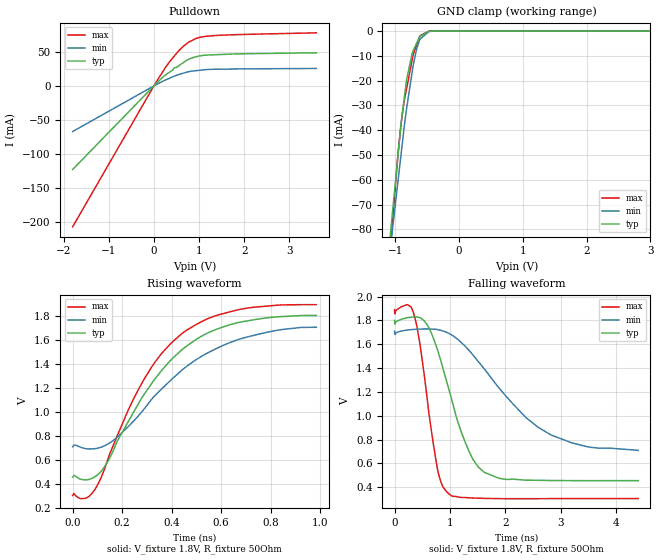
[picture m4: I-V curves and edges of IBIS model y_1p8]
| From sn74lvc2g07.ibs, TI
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|   y_1p8 Model
[Model]   y_1p8
Model_type   Open_drain
Polarity   Non-Inverting
Vmeas = 0.9
Vref = 1.8
Cref = 2pF
Rref = 1200
|   typ   min   max
|   (nom PVT)   (fast PVT)   (slow PVT)
|C_comp from frequency sweep method (F=5MHz)
C_comp   3.504e-12   3.501e-12   3.508e-12
|ON state : BUFFER OUTPUT TURNED LOW
|C_comp   7.638e-12   7.615e-12   7.652e-12
|OFF state: BUFFER IN HIGH IMPEDANCE
|C_comp   3.504e-12   3.501e-12   3.508e-12
|C_comp from LC tank measurement(L=1nH)
|Resonant Frequency(Hz)   2.600e+09   2.640e+09   2.500e+09
|C_comp   3.751e-12   3.638e-12   4.057e-12
|ON state : BUFFER OUTPUT TURNED LOW
|Resonant Frequency(Hz)   2.600e+09   2.640e+09   2.500e+09
|C_comp   3.751e-12   3.638e-12   4.057e-12
|OFF state: BUFFER IN HIGH IMPEDANCE
|Resonant Frequency(Hz)   2.720e+09   2.730e+09   2.710e+09
|C_comp   3.427e-12   3.402e-12   3.452e-12
| Where nom  PVT is Nominal Process, 1.8V, 27C
|   Fast PVT is Strong Process,  1.89V, -40C
|   Slow PVT is Weak Process,   1.71V, 125C
[Voltage Range]   1.8   1.71   1.89
|Ambient Temperature   25   85   -40
|Junction Temperature
[Temperature Range]   27   125   -40
[Pullup Reference]   1.8   1.71   1.89
[Pulldown Reference]   0   0   0
[Power Clamp Reference]   1.8   1.71   1.89
[GND Clamp Reference]   0   0   0
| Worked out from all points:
|   slope of the pulldown table from 0 to 0.27 V, typ, clamps not added: 16.1 ohm
|   GND clamp passes 1 mA (typ) near -0.53 V on its own axis
|   falling waveform, V_fixture 1.8V, R_fixture 50Ohm: 20-80 % time 533ps typ, 1.16ns min, 282ps max; typ from 1.8 V to 0.456 V
|   rising waveform, V_fixture 1.8V, R_fixture 50Ohm: 20-80 % time 278ps typ, 320ps min, 255ps max; typ from 0.457 V to 1.8 V
[Pulldown]
|   Voltage   I(typ)   I(min)   I(max)
-1.8V     -123mA     -67.12mA   -207.3mA
39.69mV   2.626mA    1.43mA     4.492mA
252mV     15.91mA    8.562mA    26.61mA
332.6mV   19.61mA    10.94mA    34.17mA
413.8mV   23.33mA    13.33mA    40.81mA
457.3mV   26.85mA    14.45mA    44.37mA
494.2mV   27.02mA    15.4mA     47.39mA
655.8mV   34.44mA    18.86mA    58.44mA
736.2mV   38.12mA    20.41mA    62.66mA
937.4mV   42.99mA    22.45mA    69.99mA
1.157V    45.34mA    24mA       73.05mA
3.6V      48.76mA    25.7mA     78.1mA
[GND Clamp]
|   Voltage   I(typ)   I(min)   I(max)
-1.8V     -317.6mA   -268.9mA   -375.6mA
-1.067V   -80.12mA   -85.85mA   -86.06mA
-958.2mV  -50.93mA   -61.3mA    -50.42mA
-907.2mV  -37.39mA   -49.82mA   -37.49mA
-863.7mV  -28.48mA   -40.04mA   -29.09mA
-820.8mV  -19.67mA   -31.39mA   -23.33mA
-718.2mV  -7.954mA   -13.99mA   -9.618mA
-661.8mV  -4.796mA   -7.109mA   -5.584mA
-610.5mV  -2.137mA   -3.249mA   -1.917mA
-470.3mV  -95.43uA   -227.8uA   -41.77uA
-383mV    -8.378uA   -33.4uA    -2.207uA
3.6V      0A         0A         0A
[POWER Clamp]
|   Voltage   I(typ)   I(min)   I(max)
-1.8V     0A         0A         0A
0V        0A         0A         0A
3.6V      0A         0A         0A
[Ramp]
R_load = 1200
|   typ   min   max
dV/dt_r   1.06682/5.72378e-09   1.00305/5.72064e-09   1.12577/5.71118e-09
dV/dt_f   1.06682/3.35081e-10   1.00306/6.32007e-10   1.12577/2.01942e-10
[Falling Waveform]
V_fixture = 1.8V
V_fixture_min = 1.71V
V_fixture_max = 1.89V
R_fixture = 50Ohm
|   Time   V(typ)   V(min)   V(max)
0s        1.8V       1.71V      1.89V
345ps     1.83V      1.725V     1.86V
455ps     1.824V     1.727V     1.613V
575ps     1.773V     1.729V     1.2V
775ps     1.554V     1.723V     551.2mV
985ps     1.216V     1.691V     342.4mV
1.345ns   701.8mV    1.549V     311.4mV
1.635ns   522.4mV    1.385V     306.5mV
2.825ns   456.6mV    839.4mV    304.7mV
4.4ns     455.8mV    709.9mV    305.4mV
[Rising Waveform]
V_fixture = 1.8V
V_fixture_min = 1.71V
V_fixture_max = 1.89V
R_fixture = 50Ohm
|   Time   V(typ)   V(min)   V(max)
0s        457.3mV    710.9mV    305.4mV
60ps      436.3mV    692.7mV    289.7mV
115ps     505.7mV    706.6mV    454mV
220ps     901.8mV    868mV      992.9mV
280ps     1.117V     1.001V     1.238V
355ps     1.332V     1.18V      1.472V
440ps     1.512V     1.344V     1.647V
545ps     1.654V     1.489V     1.773V
665ps     1.739V     1.597V     1.846V
985ps     1.8V       1.702V     1.89V
